FUNCTION_BLOCK "Main"
VERSION : 0.1
   VAR_INPUT
      in1 : Int;
      in2 : Int;
   END_VAR

   VAR_OUTPUT
      out1 : Int;
   END_VAR

   VAR_TEMP
      compResult : Bool;
   END_VAR


BEGIN
NETWORK
TITLE =

      L #in1;
      L INT#1000;
      <=I;
      = #compResult;
      CALL "__CPROVER_assume"
      (  condition                   := #compResult
      );

      L #in1;
      L INT#-1000;
      >=I;
      = #compResult;
      CALL "__CPROVER_assume"
      (  condition                   := #compResult
      );

      L #in2;
      L INT#1000;
      <=I;
      = #compResult;
      CALL "__CPROVER_assume"
      (  condition                   := #compResult
      );

      L #in2;
      L INT#-1000;
      >=I;
      = #compResult;
      CALL "__CPROVER_assume"
      (  condition                   := #compResult
      );

      L #in1;
      L #in2;
      +I;
      T #out1;
      L INT#3000;
      <I;
      = #compResult;
      CALL "__CPROVER_assert"
      (  condition                   := #compResult
      );

END_FUNCTION_BLOCK

